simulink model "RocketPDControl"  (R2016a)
settings: Solver=VariableStepAuto  StartTime=0.0  StopTime=Tf  MaxStep=1e-4  RelTol=1e-7  AbsTol=1e-6
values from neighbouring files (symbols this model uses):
  d = 0    [Section4p2_DCMotorOpenLoop.m]    (also in Section4p3_DCMotorPControl.m; Section4p4_DCMotorPIControl.m; Section4p5_RocketPDControl.m = -0.01; Section4p6_PIDSecondOrder.m = 2)
  Gden = [1 a0]    [Section4p2_DCMotorOpenLoop.m]    (also in Section4p3_DCMotorPControl.m = [J*L (J*R+b*L) (Kt*Ke+b*R)]; Section4p4_DCMotorPIControl.m; Section4p5_RocketPDControl.m = [1 a1 a0]; Section4p6_PIDSecondOrder.m = [1 a1 a0])
  Gnum = b0    (= 766.8)    [Section4p2_DCMotorOpenLoop.m]    (also in Section4p3_DCMotorPControl.m = 0.00122680374957; Section4p4_DCMotorPIControl.m; Section4p5_RocketPDControl.m = 6.32; Section4p6_PIDSecondOrder.m = 17)
  Kd = (2*zeta*wn-a1)/b0    [Section4p5_RocketPDControl.m]    (also in Section4p6_PIDSecondOrder.m = 1)
  Kp = 16    [Section4p3_DCMotorPControl.m]    (also in Section4p4_DCMotorPIControl.m = 0.002; Section4p5_RocketPDControl.m = (wn^2-a0)/b0; Section4p6_PIDSecondOrder.m = 4.94237695078; Section4p6_PIFirstOrder.m = 2)
  r = 1000    [Section4p2_DCMotorOpenLoop.m]    (also in Section4p3_DCMotorPControl.m; Section4p4_DCMotorPIControl.m; Section4p5_RocketPDControl.m = 0.1; Section4p6_PIDSecondOrder.m = 4)
  Tf = 5    [Section4p2_DCMotorOpenLoop.m]    (also in Section4p3_DCMotorPControl.m = 0.005; Section4p4_DCMotorPIControl.m = 10; Section4p5_RocketPDControl.m = 10; Section4p6_PIDSecondOrder.m = 4)
  ulim = inf    [Section4p3_DCMotorPControl.m]    (also in Section4p4_DCMotorPIControl.m; Section4p5_RocketPDControl.m)

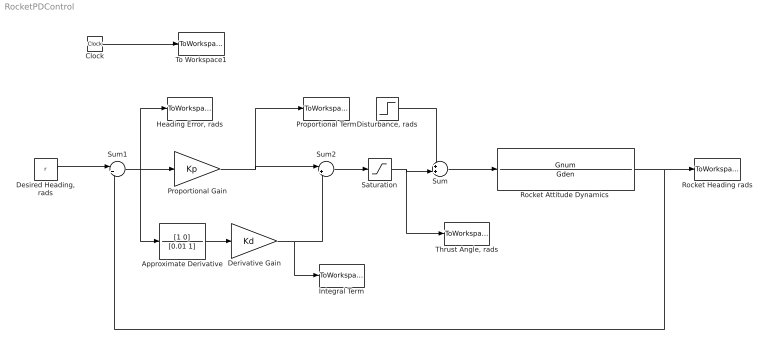
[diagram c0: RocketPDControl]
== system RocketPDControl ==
  Approximate Derivative : TransferFcn  Numerator=[1 0]  Denominator=[0.01 1]
  Clock : Clock
  Derivative Gain : Gain  Gain=Kd
  "Desired Heading, rads" : Constant  Value=r
  "Disturbance, rads" : Step  Time=Tf/2  After=d  SampleTime=0
  "Heading Error, rads" : ToWorkspace  VariableName=e  SampleTime=-1
  Integral Term : ToWorkspace  VariableName=ud  SampleTime=-1
  Proportional Gain : Gain  Gain=Kp
  Proportional Term : ToWorkspace  VariableName=up  SampleTime=-1
  "Rocket Attitude Dynamics " : TransferFcn  Numerator=Gnum  Denominator=Gden
  Rocket Heading rads : ToWorkspace  VariableName=y  SampleTime=-1
  Saturation : Saturate  UpperLimit=ulim  LowerLimit=-ulim
  Sum : Sum  Inputs=++|
  Sum1 : Sum  Inputs=|+-
  Sum2 : Sum  Inputs=|++
  "Thrust Angle, rads" : ToWorkspace  VariableName=u  SampleTime=-1
  To Workspace1 : ToWorkspace  VariableName=t  SampleTime=-1
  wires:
  Clock/1 -> To Workspace1/1
  "Disturbance, rads"/1 -> Sum/1
  Sum/1 -> "Rocket Attitude Dynamics "/1
  "Rocket Attitude Dynamics "/1 -> Sum1/2, Rocket Heading rads/1
  Sum1/1 -> Approximate Derivative/1, Proportional Gain/1, "Heading Error, rads"/1
  Saturation/1 -> Sum/2, "Thrust Angle, rads"/1
  Approximate Derivative/1 -> Derivative Gain/1
  Sum2/1 -> Saturation/1
  Derivative Gain/1 -> Integral Term/1, Sum2/2
  Proportional Gain/1 -> Proportional Term/1, Sum2/1
  "Desired Heading, rads"/1 -> Sum1/1
